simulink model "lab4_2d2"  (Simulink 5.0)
settings: Solver=FixedStepDiscrete  StartTime=0.0  StopTime=10*1e-3  FixedStep=T  RelTol=1e-3
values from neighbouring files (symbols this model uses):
  T = 1/Fsamp    (= 0.0001)    [lab4_4.m]

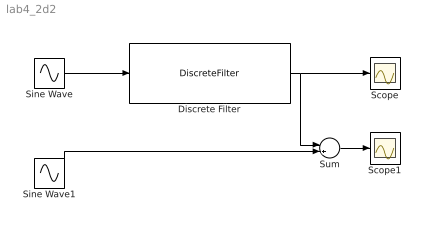
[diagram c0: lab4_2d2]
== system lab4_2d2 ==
  Discrete Filter : DiscreteFilter  Numerator="[2  1]"  Denominator="[1  -1.8*cos(pi/16)  0.81]"  SampleTime=T
  Scope : Scope
  Scope1 : Scope
  Sine Wave : Sin  Frequency=2*pi*1e3  Phase=pi/4  SampleTime=T
  Sine Wave1 : Sin  Frequency=2*pi*1e3  Phase=pi/4  SampleTime=0
  Sum : Sum  Inputs=|++
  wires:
  Discrete Filter/1 -> Scope/1, Sum/1
  Sine Wave/1 -> Discrete Filter/1
  Sum/1 -> Scope1/1
  Sine Wave1/1 -> Sum/2
